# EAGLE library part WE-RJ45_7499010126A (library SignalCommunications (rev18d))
WE-RJ45 LAN Transformer Order Code 7499010126A Design THT xBase-T 10/100 Base-T Ports 1x1 Application Standard Tab Position Vertical LED (Left-Right) Yellow-Green EMI Fingers No Details see: http://katalog.we-online.de/en/pbs/WE-LAN-RJ45 Created by Yingchun Shan 2016 (C) Wurth Elektronik
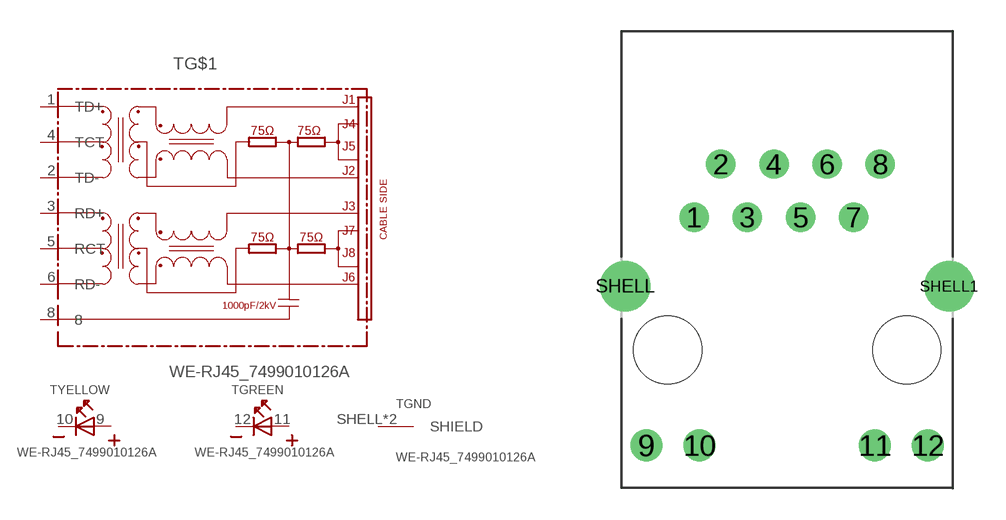
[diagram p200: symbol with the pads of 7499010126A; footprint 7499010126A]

Designator prefix T; gates G$1=7499010126A YELLOW=LED_2PIN GREEN=LED_2PIN GND=SHIELD

## WE-RJ45_7499010126A  [7499010126A]
1  G$1:TD+
2  G$1:TD-
3  G$1:RD+
4  G$1:TCT
5  G$1:RCT
6  G$1:RD-
8  G$1:8
9  YELLOW:A  pas
10  YELLOW:K  pas
11  GREEN:A  pas
12  GREEN:K  pas
SHELL  GND:SHIELD  pas
SHELL1  GND:SHIELD  pas

## Footprint 7499010126A (pad centres in mm)
drill 0.9: 1 -4.445,6.35; 2 -3.175,8.89; 3 -1.905,6.35; 4 -0.635,8.89; 5 0.635,6.35; 6 1.905,8.89; 7 3.175,6.35; 8 4.445,8.89
drill 1.02: 9 -6.73,-4.57; 10 -4.19,-4.57; 11 4.19,-4.57; 12 6.73,-4.57
drill 1.6: SHELL -7.745,3.05; SHELL1 7.745,3.05
hole 3.25 at -5.715,0
hole 3.25 at 5.715,0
